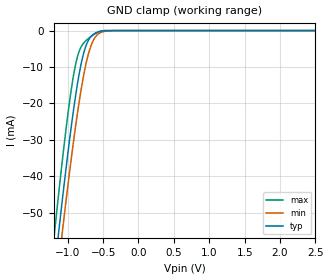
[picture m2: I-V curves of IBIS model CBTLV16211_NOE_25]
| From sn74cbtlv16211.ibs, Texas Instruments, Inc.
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[Model]   CBTLV16211_NOE_25
Model_type  Input
Vinl = 0.7
Vinh = 1.7
| variable   typ   min   max
C_comp   2.41pF   1.85pF   2.89pF
[Temperature Range]   40   100   -40
| Ambient temperature   25   85   -40
[Voltage range]   2.5   2.3   2.7
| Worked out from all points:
|   GND clamp passes 1 mA (typ) near -0.63 V on its own axis
[GND Clamp]
| CBTLV16211_NOE_25
|   Voltage   I(typ)   I(min)   I(max)
-2.5V     -335.6mA   -337.2mA   -335.7mA
-1.19V    -66.45mA   -74.91mA   -56.19mA
-1.14V    -57.6mA    -66.24mA   -47.05mA
-1.115V   -53.25mA   -61.97mA   -42.58mA
-1.07V    -45.57mA   -54.41mA   -34.77mA
-960mV    -27.97mA   -36.8mA    -17.62mA
-870mV    -15.62mA   -23.79mA   -7.765mA
-755mV    -4.939mA   -10.4mA    -2.998mA
-680mV    -1.864mA   -4.686mA   -1.771mA
-615mV    -753.8uA   -1.929mA   -884.8uA
-395mV    -3.656uA   -52.45uA   -106.2nA
2.5V      1.122nA    59.66nA    7.278pA
